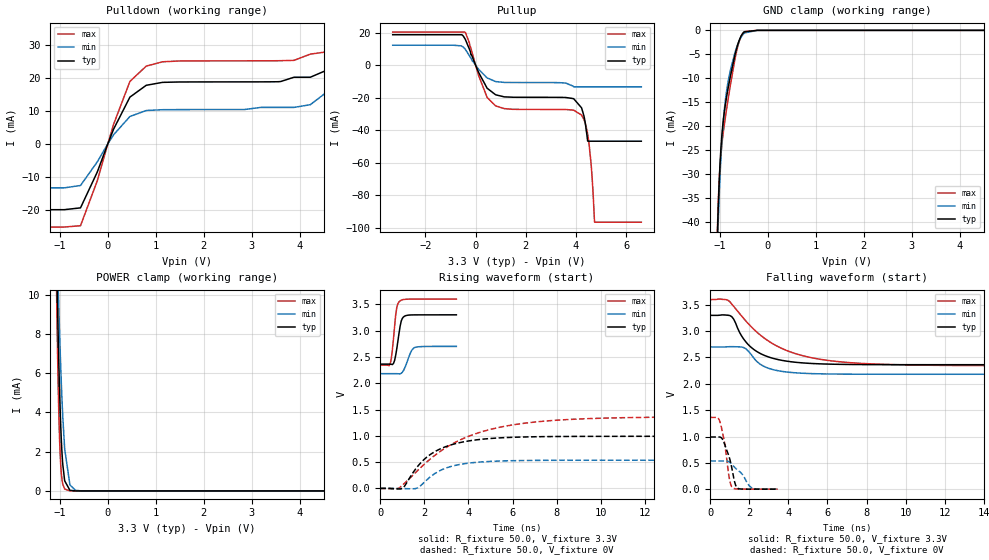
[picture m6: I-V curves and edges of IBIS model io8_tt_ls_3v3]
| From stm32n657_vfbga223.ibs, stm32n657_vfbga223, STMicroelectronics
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[Model]   io8_tt_ls_3v3
Model_type I/O
Polarity   Non-Inverting
Enable   Active-Low
| CAP_THRESHOLD on pad IOTT is "UDTCAPC" :
| Rising=30.0% of vddiov33m   Falling=70.0% of vddiov33m
| C_comp min and max val. don't necessarily correlate with the min and max pvt
| but are the smallest and greatest pad capacitance found.
| var   typ   min   max
C_comp   1.01863pF  1.01060pF  1.02128pF
|C_comp_pullup   495.66500fF  479.36000fF  510.70500fF
|C_comp_pulldown   522.96000fF  531.23929fF  510.57500fF
Vinl = 1.35V
Vinh = 1.8V
Vmeas = 1.65V   | Reference voltage for timing measurements
Cref  = 50.0pF   | Timing specification test load capacitance value
Rref  = 1.0MOhm   | Timing specification test load resistance value
Vref  = 1.815V   | Timing specification test load voltage
[Model Spec]
| TIME_THRESHOLD on pin ZIV08M is "CMOS" :
| Rising=50.0% of vddv08m   Falling=50.0% of vddv08m
Vinl 1.08570V 868.70000mV 1.21270V
Vinh 1.55630V 1.26230V 1.70930V
| variable   typ   min   max
[Temperature Range] 25.0 125.0 -40.0
| variable   typ   min   max
[Voltage Range] 3.3V 2.7V 3.6V
| variable   typ   min   max
[POWER Clamp Reference] 3.3V 2.7V 3.6V
| variable   typ   min   max
[GND Clamp Reference] 0V 0V 0V
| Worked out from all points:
|   slope of the pulldown table from 0 to 0.495 V, typ, clamps not added: 34.1 ohm
|   slope of the pullup table from 0 to 0.495 V, typ, clamps not added: 33.8 ohm
|   GND clamp passes 1 mA (typ) near -0.55 V on its own axis
|   POWER clamp passes 1 mA (typ) near -0.92 V on its own axis
|   rising waveform, R_fixture 50.0, V_fixture 3.3V: 20-80 % time 208ps typ, 287ps min, 179ps max; typ from 2.36 V to 3.3 V
|   falling waveform, R_fixture 50.0, V_fixture 3.3V: 20-80 % time 1.37ns typ, 1.06ns min, 2.71ns max; typ from 3.3 V to 2.36 V
|   rising waveform, R_fixture 50.0, V_fixture 0V: 20-80 % time 1.63ns typ, 1.34ns min, 3.19ns max; typ from 0 V to 0.99 V
|   falling waveform, R_fixture 50.0, V_fixture 0V: 20-80 % time 418ps typ, 701ps min, 329ps max; typ from 0.991 V to 0 V
[POWER Clamp]
-3.3V     1.353A     318.4mA    2.015A
-1.07V    12.07mA    13.62mA    10.38mA
-1.06V    10.79mA    12.68mA    8.745mA
-1.05V    9.571mA    11.76mA    7.253mA
-1.03V    7.341mA    9.999mA    4.748mA
-1V       4.588mA    7.595mA    2.215mA
-980mV    3.183mA    6.171mA    1.238mA
-950mV    1.704mA    4.337mA    481.8uA
-900mV    515.5uA    2.141mA    93.34uA
-790mV    29.45uA    301.7uA    4.884uA
-670mV    1.871uA    28.97uA    2.19uA
6.6V      0A         0A         0A
[GND Clamp]
-3.3V     -3.772A    -3.743A    -3.788A
-1.05V    -42.34mA   -45.44mA   -41.2mA
-1.04V    -38.9mA    -42mA      -37.88mA
-1.03V    -35.84mA   -38.88mA   -35.06mA
-1V       -28.57mA   -31.07mA   -28.88mA
-970mV    -23.48mA   -25.09mA   -24.97mA
-920mV    -18.07mA   -17.99mA   -20.63mA
-860mV    -13.91mA   -12.68mA   -16.46mA
-780mV    -9.536mA   -8.318mA   -11.38mA
-650mV    -3.744mA   -3.567mA   -4.327mA
-490mV    -324.2uA   -555.2uA   -259.7uA
6.6V      214nA      4.276uA    223.3nA
| variable   typ   min   max
[Pullup Reference] 3.3V 2.7V 3.6V
| variable   typ   min   max
[Pulldown Reference] 0V 0V 0V
[Pullup]
-3.3V     18.7mA     12.27mA    20.34mA
-430mV    16.42mA    10.12mA    20.31mA
460mV     -14.22mA   -7.865mA   -19.9mA
800mV     -18.26mA   -10.12mA   -25.1mA
3.88V     -20.57mA   -12.91mA   -27.66mA
4.22V     -26.27mA   -13.36mA   -30.72mA
4.35V     -33.99mA   -13.36mA   -34.99mA
4.46V     -46.57mA   -13.36mA   -42.29mA
4.52V     -46.82mA   -13.36mA   -48.77mA
4.63V     -46.82mA   -13.36mA   -66.94mA
4.74V     -46.82mA   -13.36mA   -96.67mA
6.6V      -46.82mA   -13.36mA   -96.67mA
[Pulldown]
-3.3V     -19.95mA   -13.34mA   -25.2mA
-570mV    -19.4mA    -12.62mA   -24.8mA
-220mV    -8.542mA   -5.471mA   -11.2mA
120mV     4.438mA    2.727mA    5.906mA
460mV     14.14mA    8.269mA    18.88mA
800mV     17.71mA    10.08mA    23.52mA
3.88V     20.15mA    11.02mA    25.27mA
4.22V     20.15mA    11.84mA    27.14mA
4.56V     22.27mA    15.62mA    27.84mA
4.9V      31.19mA    28.06mA    34.85mA
5.25V     61.06mA    66.66mA    59.35mA
6.6V      396.6mA    415.2mA    364.3mA
[Ramp]
dV/dt_r 594.29853mV/1.62814ns 321.45416mV/1.33802ns 817.90922mV/3.18552ns
dV/dt_f 562.25346mV/1.36611ns 311.02027mV/1.0574ns 753.5197mV/2.71333ns
R_load = 50.0
| Removed startup time: 0s 0s 0s  .
| Removed end time: 3.45ns.
[Rising Waveform]
R_fixture   = 50.0
V_fixture   = 3.3V
V_fixture_min = 2.7V
V_fixture_max = 3.6V
0s        2.363V     2.182V     2.344V
450ps     2.363V     2.182V     2.364V
500ps     2.36V      2.182V     2.466V
600ps     2.377V     2.182V     2.853V
750ps     2.66V      2.181V     3.444V
900ps     3.083V     2.177V     3.566V
1.05ns    3.259V     2.239V     3.591V
1.4ns     3.298V     2.605V     3.599V
1.55ns    3.299V     2.675V     3.599V
3.45ns    3.3V       2.7V       3.6V
| Removed startup time: 0s 0s 0s  .
| Removed end time: 24.9ns.
[Falling Waveform]
R_fixture   = 50.0
V_fixture   = 3.3V
V_fixture_min = 2.7V
V_fixture_max = 3.6V
0s        3.3V       2.7V       3.6V
800ps     3.306V     2.701V     3.598V
1.1ns     3.275V     2.706V     3.515V
1.8ns     2.806V     2.671V     3.203V
2.4ns     2.61V      2.419V     2.977V
2.8ns     2.535V     2.323V     2.858V
4.2ns     2.416V     2.214V     2.593V
5.9ns     2.376V     2.188V     2.45V
10.4ns    2.363V     2.182V     2.357V
24.9ns    2.363V     2.182V     2.344V
| Removed startup time: 0s 0s 0s  .
| Removed end time: 24.9ns.
[Rising Waveform]
R_fixture   = 50.0
V_fixture   = 0V
V_fixture_min = 0V
V_fixture_max = 0V
0s        541.8nV    3.002uV    641.8nV
700ps     -6.768mV   -142.6uV   -14.51mV
1ns       -1.762mV   -2.048mV   60.21mV
1.6ns     367.7mV    -3.319mV   301.8mV
2ns       555mV      118.4mV    461.5mV
3ns       798.7mV    389.9mV    780.7mV
4.5ns     929.8mV    500.6mV    1.064V
6.4ns     976.5mV    529.5mV    1.232V
11.1ns    990.2mV    535.7mV    1.345V
24.9ns    990.5mV    535.8mV    1.363V
| Removed startup time: 0s 0s 0s  .
| Removed end time: 3.45ns.
[Falling Waveform]
R_fixture   = 50.0
V_fixture   = 0V
V_fixture_min = 0V
V_fixture_max = 0V
0s        990.5mV    535.8mV    1.363V
350ps     990.5mV    535.8mV    1.362V
500ps     988.9mV    535.8mV    1.273V
750ps     839.3mV    535.9mV    833.6mV
1ns       569.5mV    511.3mV    153.9mV
1.15ns    310.9mV    454.3mV    24.45mV
1.3ns     72.26mV    395.5mV    5.699mV
1.45ns    9.919mV    346.5mV    2.491mV
2.15ns    553uV      22.66mV    720uV
3.45ns    149.6uV    134.8uV    245.6uV
